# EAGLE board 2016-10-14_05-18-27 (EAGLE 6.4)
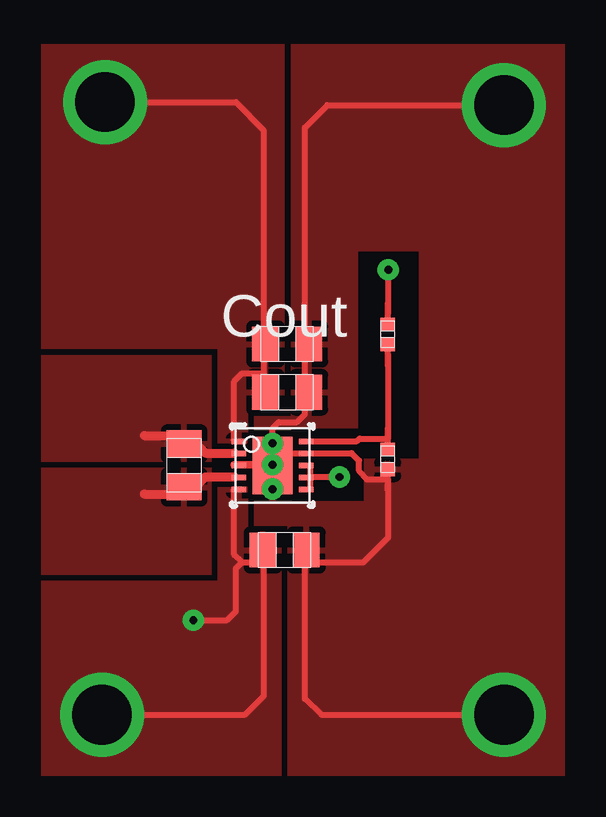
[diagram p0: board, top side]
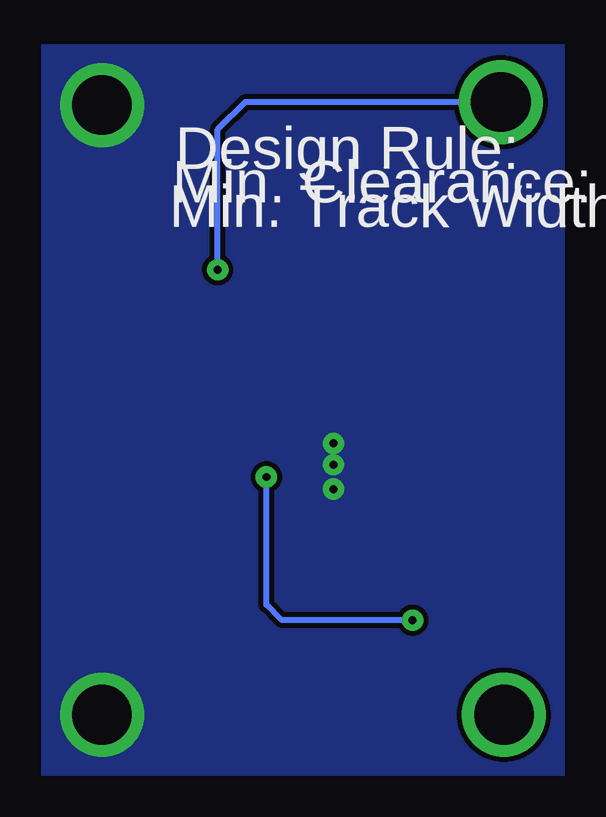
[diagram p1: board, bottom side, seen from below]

No outline drawn. Coordinates in mm, seen from the top.
Copper layers ((1*2)+(15*16)): TOP / INTERNAL1 / layer 15 / BOTTOM

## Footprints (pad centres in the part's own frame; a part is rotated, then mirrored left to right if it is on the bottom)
0805 = smd 1.118 x 1.448: 1 -0.902,0; 2 0.902,0
TP-1502 = drill 0.813 round: 1 0,0
0402 = smd 0.559 x 0.61: 1 -0.419,0; 2 0.419,0
DRC0010J = smd 0.6 x 0.24: 1 -1.4,1; 2 -1.4,0.5; 3 -1.4,0; 4 -1.4,-0.5; 5 -1.4,-1; 6 1.4,-1; 7 1.4,-0.5; 8 1.4,0; 9 1.4,0.5; 10 1.4,1 | smd 1.65 x 2.4: 11 0,0

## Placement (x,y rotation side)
Cin  [0805]  36.58,36.07 0 top
Cout_1  [0805]  36.68,42.65 0 top
Cout_2  [0805]  36.68,44.65 0 top
GND  [TP-1502]  45.69,29.18 0 top
GND1  [TP-1502]  45.69,54.58 0 top
L1  [0805]  32.38,39.6 90 top
Rfbb  [0402]  40.87,39.85 270 top
Rfbt  [0402]  40.87,45.06 270 top
U1  [DRC0010J]  36.07,39.6 0 top
VIN  [TP-1502]  28.93,29.18 0 top
VOUT  [TP-1502]  29.06,54.74 0 top

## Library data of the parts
Cin = ultra-librarian; RefDes: Cin; Type: LMK212BJ106KG-T
Cout_1 Cout_2 = ultra-librarian
GND = ultra-librarian; RefDes: GND; Type: TP-1502
GND1 = ultra-librarian; RefDes: GND1; Type: TP-1502
L1 = ultra-librarian; RefDes: L1; Type: LQM21PN1R5MC0D
Rfbb = ultra-librarian; RefDes: Rfbb; Type: CRCW0402178KFKED
Rfbt = ultra-librarian; RefDes: Rfbt; Type: CRCW04021M00FKED
U1 = ultra-librarian; RefDes: U1; Type: TPS63000DRCR
VIN = ultra-librarian; RefDes: VIN; Type: TP-1502
VOUT = ultra-librarian; RefDes: VOUT; Type: TP-1502

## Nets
0: Cin.2 Cout_1.2 Cout_2.2 GND1.1 GND.1 Rfbb.2 U1.3 U1.9 U1.11
3: Rfbb.1 Rfbt.2 U1.10
6: Cout_1.1 Cout_2.1 Rfbt.1 U1.1 VOUT.1
7: L1.1 U1.4
10: L1.2 U1.2
11: Cin.1 U1.5 U1.6 U1.7 U1.8 VIN.1

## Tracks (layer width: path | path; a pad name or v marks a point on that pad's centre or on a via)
0  (via drill 0.33 pad 0.89, 2.49 pad 3.48)
  TOP 0.254: v36.07,40.51 36.07,41.15 36.32,41.4 37.08,41.4 37.41,41.73 37.41,53.67 38.35,54.61 v45.72,54.61 | v36.07,39.62 36.7,39.62 36.7,40.11 37.64,40.11 39.37,40.11 39.67,39.8 39.67,39.37 40.01,39.01 40.89,39.01 40.89,36.6 39.85,35.56 37.41,35.56 37.41,29.87 38.1,29.21 v45.72,29.21 | 40.88,38.53 40.88,39.47
  TOP 0.305: 34.47,39.62 v36.07,39.62
  other vias: 36.07,38.61
  pour TOP (rank 6): 35.31,39.62 36.83,39.62 36.83,38.1 39.88,38.1 39.88,39.88 42.16,39.88 42.16,48.51 39.62,48.51 39.62,41.15 36.83,41.15 36.83,39.75 35.31,39.75 35.31,41.66 36.83,41.66 36.83,57.15 48.26,57.15 48.26,26.67 36.7,26.67 36.7,37.08 35.31,37.08
  pour BOTTOM (rank 5): 26.42,57.15 48.26,57.15 48.26,26.67 26.42,26.67
3
  TOP 0.254: 40.89,44.22 40.89,40.72 39.7,40.72 39.6,40.62 37.64,40.62 | 40.88,40.23 40.88,41.17 | 40.88,43.74 40.88,44.68
6  (via drill 0.33 pad 0.89, 2.49 pad 3.48)
  TOP 0.254: v29.08,54.74 34.54,54.74 35.71,53.54 35.71,43.43 34.8,43.43 34.47,43.1 34.47,40.62 | 40.89,45.92 v40.89,47.75 | 40.88,45.44 40.88,46.38
  BOTTOM 0.254: v40.89,47.75 40.89,53.59 39.75,54.74 v29.08,54.74
  pour TOP (rank 4): 33.78,40.51 35.05,40.51 35.05,41.91 36.58,41.91 36.58,57.15 26.42,57.15 26.42,44.45 33.78,44.45
7
  TOP 0.381: 30.73,38.41 32.56,38.41 33.27,39.12 34.47,39.12
  pour TOP: 33.53,39.5 26.42,39.5 26.42,35.05 33.53,35.05
10
  TOP 0.381: 34.47,40.11 33.27,40.11 32.56,40.84 30.73,40.84
  pour TOP (rank 2): 33.53,39.75 33.53,44.2 26.42,44.2 26.42,39.75
11  (via drill 0.33 pad 0.89, 2.49 pad 3.48)
  TOP 0.254: v32.77,33.15 34.16,33.15 34.54,33.53 34.54,35.31 34.8,35.56 | 34.8,35.56 34.47,35.87 34.47,38.61 | 34.8,35.56 35.71,35.56 35.71,30 34.92,29.21 v28.96,29.21 | 37.64,39.12 | 37.64,39.12 v38.86,39.12 | 37.64,38.61 37.64,39.12 | 37.64,39.12 37.64,39.62
  BOTTOM 0.254: v38.86,39.12 38.86,33.78 38.23,33.15 v32.77,33.15
  pour TOP (rank 3): 33.78,38.73 35.05,38.73 35.05,36.83 36.45,36.83 36.45,26.67 26.42,26.67 26.42,34.8 33.78,34.8

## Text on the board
ASSYNOTES: Cout
bDocu: Design Rule: | Min. Clearance: 10mil | Min. Track Width: 10mil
